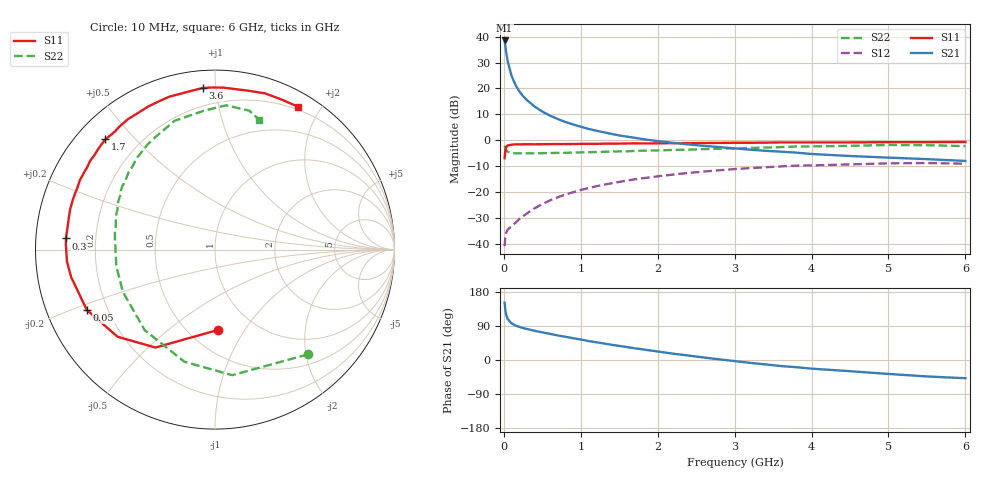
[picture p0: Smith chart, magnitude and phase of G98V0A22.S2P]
! SIEMENS Small Signal Semiconductors
! BFG235
! Si NPN RF Bipolar Junction Transistor in SOT223
! VCE = 8 V  IC = 220 mA
! Common Emitter S-Parameters:  July  1994
# GHz  S  MA  R  50
!  f  S11  S21  S12  S22
! GHz  MAG  ANG  MAG  ANG  MAG  ANG  MAG  ANG
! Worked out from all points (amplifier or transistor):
!   40 points, 10 MHz to 6 GHz, reference 50 ohm
!   highest |S21| = 38.6 dB at 10 MHz (marker M1)
!   |S21| within 3 dB of that: start of sweep to 23.52 MHz
!   unconditionally stable (mu >= 1): 430.8 MHz to 1.526 GHz
!   at 200 MHz: K = 0.82, MSG = 24.7 dB, |S12| = -30.5 dB
!   at 1.5 GHz: K = 1.00, MAG = 8.6 dB, |S12| = -16.1 dB
!   at 6 GHz: K = 0.90, MSG = 0.5 dB, |S12| = -9.1 dB
!   S11 on the Smith chart (normalised r, x): 10 MHz: 0.68, -0.77; 50 MHz: 0.12, -0.22; 300 MHz: 0.09, +0.04; 1.7 GHz: 0.08, +0.41; 3.6 GHz: 0.09, +0.92; 6 GHz: 0.17, +1.72
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0.01  0.4484 -88.1  84.66 151.1  0.0089 60.3  0.7805 -48.4
0.02  0.6386 -121.3  65.53 131.8  0.0138 46.8  0.7062 -82.2
0.03  0.7283 -138.2  50.84 120.2  0.0162 39.5  0.6475 -105.3
0.05  0.7894 -154.8  33.49 108.1  0.0186 33.5  0.5954 -131.2
0.1  0.8161 -169.2  17.6 96.7  0.0216 37.7  0.5647 -155.4
0.15  0.8275 -175.4  11.8 91.0  0.0251 44.9  0.5555 -165.5
0.2  0.8281 -178.8  8.823 87.5  0.0297 49.6  0.5577 -170.7
0.25  0.8312 178.2  7.107 84.3  0.0337 53.8  0.5543 -174.4
0.3  0.8329 175.7  5.933 81.9  0.0383 56.5  0.5552 -177.5
0.4  0.831 171.4  4.462 77.1  0.048 59.3  0.5549 178.4
0.5  0.8334 167.8  3.564 72.8  0.0582 60.8  0.5593 175.0
0.6  0.8376 164.6  2.977 69.1  0.0683 60.9  0.5635 171.9
0.8  0.8401 158.3  2.246 61.3  0.0886 59.7  0.568 166.6
1.1  0.8468 149.5  1.649 50.0  0.1183 55.9  0.5847 159.8
1.4  0.8532 142.1  1.319 40.2  0.1462 51.0  0.6018 153.7
1.7  0.8658 134.8  1.109 30.9  0.1744 45.7  0.6187 148.1
2.2  0.8738 123.7  0.886 16.7  0.2157 36.4  0.6466 138.0
3.2  0.8893 102.5  0.655 -7.5  0.2873 17.1  0.7049 119.4
3.6  0.9029 94.4  0.598 -15.9  0.31 8.7  0.7334 111.1
4.5  0.9036 79.1  0.493 -29.5  0.3396 -7.6  0.7757 94.7
5.5  0.9148 65.8  0.429 -43.4  0.3604 -25.8  0.7971 76.1
6  0.9203 59.9  0.396 -48.1  0.3502 -32.7  0.7651 71.3
